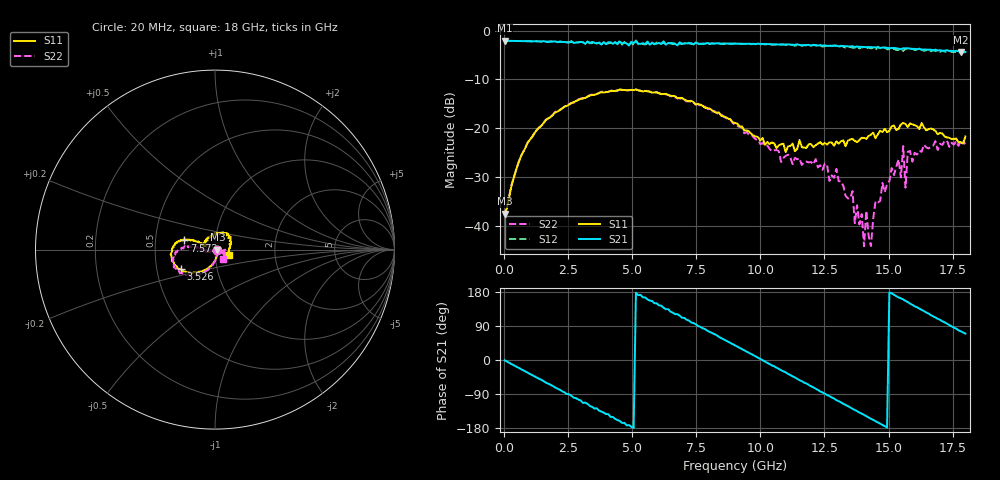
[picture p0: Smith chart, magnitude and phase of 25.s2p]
!Agilent Technologies,N5230A,US43500223,A.07.50.48
!Agilent N5230A: A.07.50.48
!Date: Saturday, January 16, 2016 17:24:41
!Correction: S11(Full 2 Port(1,2))
!S21(Full 2 Port(1,2))
!S12(Full 2 Port(1,2))
!S22(Full 2 Port(1,2))
!S2P File: Measurements: S11, S21, S12, S22:
# Hz S  dB  R 50
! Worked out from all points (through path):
!   201 points, 20 MHz to 18 GHz, reference 50 ohm
!   highest |S21| = -2.09 dB at 20 MHz (marker M1); lowest = -4.4 dB at 17.82 GHz (marker M2)
!   group delay of S21, straight-line fit = 100 ps
!   lowest |S11| = -37.5 dB at 20 MHz (marker M3), VSWR 1.03, Z = 51.3 - j0.0534 ohm
!   |S11| at or under -10 dB: start of sweep to end of sweep
!   |S22| runs from -44.2 to -12.0 dB; largest |S21 - S12| = 0.082
!   S11 on the Smith chart (normalised r, x): 20 MHz: 1.03, -0.00; 3.526 GHz: 0.67, -0.15; 7.572 GHz: 0.71, +0.07; 18 GHz: 1.16, -0.07
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2e7  -37.52 -2.2  -2.09 -0.8  -2.09 -0.8  -38.04 -2.0
9.19e8  -22.98 -94.5  -2.15 -33.5  -2.16 -33.8  -22.91 -92.5
3.0766e9  -13.87 -142.6  -2.39 -113.2  -2.37 -112.8  -13.95 -134.9
3.5261e9  -13.15 -150.1  -2.51 -128.1  -2.35 -128.6  -13.15 -141.0
5.1443e9  -12.09 -174.1  -2.14 177.4  -2.03 175.5  -12.01 -164.0
6.0433e9  -12.85 173.1  -2.53 144.0  -2.69 140.5  -12.83 -172.4
7.5716e9  -15.01 163.3  -2.67 89.3  -2.73 87.7  -15.10 176.9
9.01e9  -18.92 156.8  -2.66 38.5  -2.69 35.1  -19.30 173.8
1.03585e10  -23.26 159.8  -2.76 -10.4  -2.78 -14.1  -24.23 -178.4
1.20666e10  -23.90 153.9  -2.93 -72.1  -2.92 -76.6  -27.42 -164.8
1.35949e10  -22.21 117.4  -3.21 -128.9  -3.52 -134.5  -32.88 -161.0
1.40444e10  -21.98 99.9  -3.37 -144.9  -3.49 -151.6  -44.17 -127.1
1.41343e10  -22.19 99.0  -3.40 -148.2  -3.60 -153.5  -36.91 -69.9
1.43141e10  -21.32 95.7  -3.39 -154.9  -3.65 -158.5  -44.16 13.4
1.44939e10  -22.07 86.9  -3.41 -161.6  -3.96 -166.0  -34.95 -37.1
1.50333e10  -20.55 73.7  -3.62 178.4  -3.80 172.8  -30.89 -5.3
1.54828e10  -19.24 58.6  -3.79 162.7  -3.73 157.5  -30.07 0.9
1.55727e10  -18.92 51.7  -3.61 159.8  -4.18 155.3  -23.65 -18.1
1.56626e10  -19.14 53.5  -3.66 156.0  -3.71 152.3  -32.16 -32.3
1.57525e10  -19.77 50.3  -3.61 152.9  -3.74 146.4  -24.83 -0.3
1.78202e10  -22.86 -17.4  -4.40 75.7  -4.62 69.3  -22.60 -39.6
1.8e10  -21.70 -22.7  -4.37 69.6  -4.48 62.1  -23.26 -47.5
